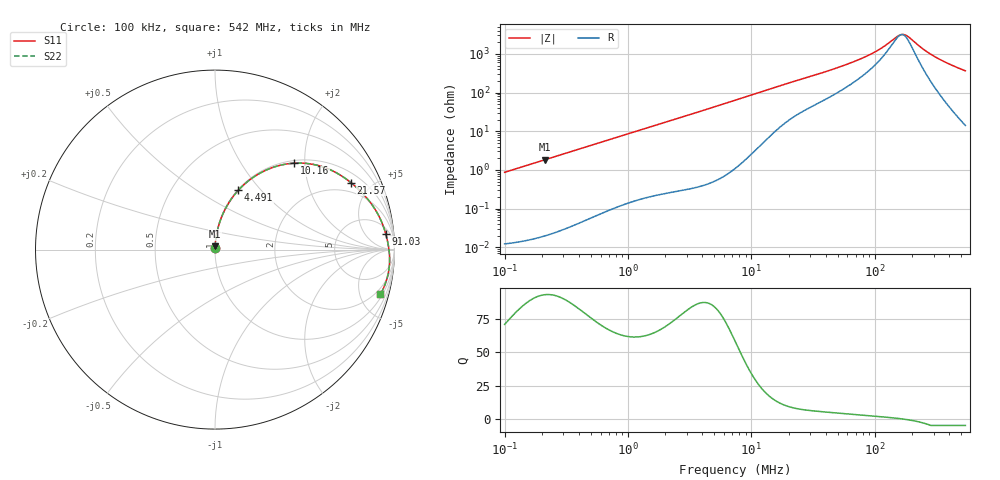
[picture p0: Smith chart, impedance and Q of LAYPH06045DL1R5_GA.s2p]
! LAYPH06045DL1R5_GA  S-PARAMETER MODEL  ( General Type )
! Model Generated by TAIYO YUDEN Corporation (http://www.ty-top.com)
! Version 2.0
! TAIYO YUDEN Control No. 180914NI43SB-FBB
! Copyright(c) 2018 TAIYO YUDEN CO.,LTD. All Rights Reserved.
! Product Description (link to TY-COMPAS)
! https://ds.yuden.co.jp/TYCOMPAS/or/detail?pn=LAYPH06045DL1R5NGA&u=M
! Products Name : Inductors
! Characteristics :
!  Inductance : 1.5 uH , SRF(min) : -Hz , DC Resistance(max) : 0.013 Ohm
!  Rated Current : Saturation :5.5 A , Temp Rise : 3.2 A (25 degC)
!  Case Size : 6.3 x 6.0 / 0.248 x 0.236 [mm/inch] , Thickness : 4.5 / 0.177 [mm/inch]
!  (Conditions: Temperature = 25 degC , DC Bias Current/Voltage = 0A / 0V)
! External Node Assignments :
!  1  o---GGG---o  2
! GND o---------o GND
! Frequency Range : 0.1MHz  -  542.002916MHz  [ 402 STEP ]
# MHz S RI R 50
! Freq[MHz].  S11 Real  S11 Imag  S21 Real  S21 Imag  S12 Real  S12 Imag  S22 Real  S22 Imag
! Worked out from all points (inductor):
!   401 points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, 100 kHz to 542 MHz, reference 50 ohm
!   read as one part in series: L = 1.38 uH near 104.4 kHz
!   highest Q = 93.4 at 212.2 kHz (marker M1), where L = 1.38 uH
!   self-resonance near 164 MHz
!   S11 on the Smith chart (normalised r, x): 100 kHz: 1.00, +0.02; 4.491 MHz: 1.01, +0.76; 10.16 MHz: 1.05, +1.77; 21.57 MHz: 1.45, +3.76; 91.03 MHz: 9, +17; 542 MHz: 1.28, -7.29
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0.1  0.000197 0.00866  0.9998 -0.00866  0.9998 -0.00866  0.000197 0.00866
0.21219  0.000534 0.0184  0.9995 -0.0184  0.9995 -0.0184  0.000534 0.0184
0.422129  0.00178 0.0364  0.9982 -0.0364  0.9982 -0.0364  0.00178 0.0364
0.935062  0.00764 0.0794  0.9924 -0.0794  0.9924 -0.0794  0.00764 0.0794
1.78193  0.0246 0.1474  0.9754 -0.1474  0.9754 -0.1474  0.0246 0.1474
2.984906  0.0628 0.2365  0.9372 -0.2365  0.9372 -0.2365  0.0628 0.2365
4.490511  0.13 0.3306  0.87 -0.3306  0.87 -0.3306  0.13 0.3306
7.362085  0.289 0.4448  0.711 -0.4448  0.711 -0.4448  0.289 0.4448
10.16309  0.4406 0.4815  0.5594 -0.4815  0.5594 -0.4815  0.4406 0.4815
14.02978  0.5988 0.4614  0.4012 -0.4614  0.4012 -0.4614  0.5988 0.4614
21.56508  0.7571 0.3732  0.2429 -0.3732  0.2429 -0.3732  0.7571 0.3732
31.0775  0.8423 0.2909  0.1577 -0.2909  0.1577 -0.2909  0.8423 0.2909
56.73175  0.9228 0.1671  0.0772 -0.1671  0.0772 -0.1671  0.9228 0.1671
91.03246  0.9515 0.0874  0.0485 -0.0874  0.0485 -0.0874  0.9515 0.0874
110.4616  0.9588 0.0584  0.0412 -0.0584  0.0412 -0.0584  0.9588 0.0584
131.1872  0.964 0.0333  0.036 -0.0333  0.036 -0.0333  0.964 0.0333
159.1866  0.9687 0.00455  0.0313 -0.00455  0.0313 -0.00455  0.9687 0.00455
177.248  0.9707 -0.012  0.0293 0.012  0.0293 0.012  0.9707 -0.012
250.0008  0.9727 -0.0706  0.0273 0.0706  0.0273 0.0706  0.9727 -0.0706
303.3587  0.9693 -0.1088  0.0307 0.1088  0.0307 0.1088  0.9693 -0.1088
401.1544  0.9551 -0.1718  0.0449 0.1718  0.0449 0.1718  0.9551 -0.1718
542.0029  0.9217 -0.25  0.0783 0.25  0.0783 0.25  0.9217 -0.25
